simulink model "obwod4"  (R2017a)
settings: Solver=VariableStepAuto  StartTime=0.0  StopTime=100.0  RelTol=1e-6
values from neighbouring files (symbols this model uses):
  A = [0,1,0,0    [obwod4m.m]
  B = [0;dx5;0;-ex5]    [obwod4m.m]
  C = [0,1,0,0    [obwod4m.m]
  D = [0;0]    [obwod4m.m]
  dx1 = w1/(1-K1*K2)    (= 0.616649537513)    [obwod4m.m]    (also in cz1.m; cz1m.m; obwod1m.m; obwod2m.m)
  dx2 = 1/(T1*(1-K1*K2))    (= 1.02774922919)    [obwod4m.m]    (also in cz1.m; cz1m.m; obwod1m.m; obwod2m.m = 0.0513874614594)
  dx3 = (w2*K1)/(1-K1*K2)    (= 0.172045220966)    [obwod4m.m]    (also in cz1.m; cz1m.m; obwod1m.m; obwod2m.m)
  dx4 = K1/(T2*(1-K1*K2))    (= 0.277492291881)    [obwod4m.m]    (also in cz1.m; cz1m.m; obwod1m.m; obwod2m.m = 0.013874614594)
  dx5 = 1/(L1*(1-K1*K2))    (= 1.02774922919)    [obwod4m.m]    (also in cz1.m; cz1m.m; obwod1m.m; obwod2m.m)
  ex1 = (w2*K2)/(1-K1*K2)    (= 0.0637204522097)    [obwod4m.m]    (also in cz1.m; cz1m.m; obwod1m.m; obwod2m.m)
  ex2 = K2/(T1*(1-K1*K2))    (= 0.102774922919)    [obwod4m.m]    (also in cz1.m; cz1m.m; obwod1m.m; obwod2m.m = 0.00513874614594)
  ex3 = w2/(1-K1*K2)    (= 0.637204522097)    [obwod4m.m]    (also in cz1.m; cz1m.m; obwod1m.m; obwod2m.m)
  ex4 = 1/(T2*(1-K1*K2))    (= 1.02774922919)    [obwod4m.m]    (also in cz1.m; cz1m.m; obwod1m.m; obwod2m.m = 0.0513874614594)
  ex5 = (K2*1)/(L1*(1-K1*K2))    (= 0.102774922919)    [obwod4m.m]    (also in cz1.m; cz1m.m; obwod1m.m; obwod2m.m)

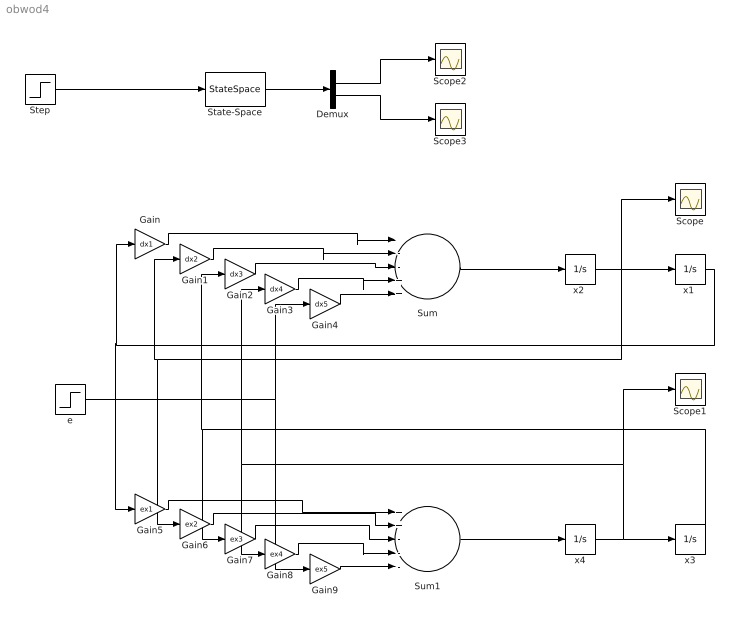
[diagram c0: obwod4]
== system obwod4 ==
  Demux : Demux  Outputs=2
  Gain : Gain  Gain=dx1
  Gain1 : Gain  Gain=dx2
  Gain2 : Gain  Gain=dx3
  Gain3 : Gain  Gain=dx4
  Gain4 : Gain  Gain=dx5
  Gain5 : Gain  Gain=ex1
  Gain6 : Gain  Gain=ex2
  Gain7 : Gain  Gain=ex3
  Gain8 : Gain  Gain=ex4
  Gain9 : Gain  Gain=ex5
  Scope{,1..3} (4 alike) : Scope
  State-Space : StateSpace  A=A  B=B  C=C  D=D  X0=0
  Step : Step  Time=0  After=10  SampleTime=0
  Sum : Sum  Inputs=|--+++
  Sum1 : Sum  Inputs=++---
  e : Step  Time=0  After=10  SampleTime=0
  "x1 " : Integrator
  "x2 " : Integrator
  x3 : Integrator
  x4 : Integrator
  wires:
  Sum/1 -> "x2 "/1
  "x2 "/1 -> Scope/1, Gain6/1, Gain1/1, "x1 "/1
  Gain4/1 -> Sum/5
  Gain3/1 -> Sum/4
  Gain2/1 -> Sum/3
  Gain1/1 -> Sum/2
  Gain/1 -> Sum/1
  "x1 "/1 -> Gain5/1, Gain/1
  Sum1/1 -> x4/1
  x4/1 -> Gain8/1, Gain3/1, Scope1/1, x3/1
  e/1 -> Gain4/1, Gain9/1
  Gain9/1 -> Sum1/5
  Gain8/1 -> Sum1/4
  Gain7/1 -> Sum1/3
  Gain6/1 -> Sum1/2
  Gain5/1 -> Sum1/1
  x3/1 -> Gain7/1, Gain2/1
  State-Space/1 -> Demux/1
  Demux/1 -> Scope2/1
  Demux/2 -> Scope3/1
  Step/1 -> State-Space/1
